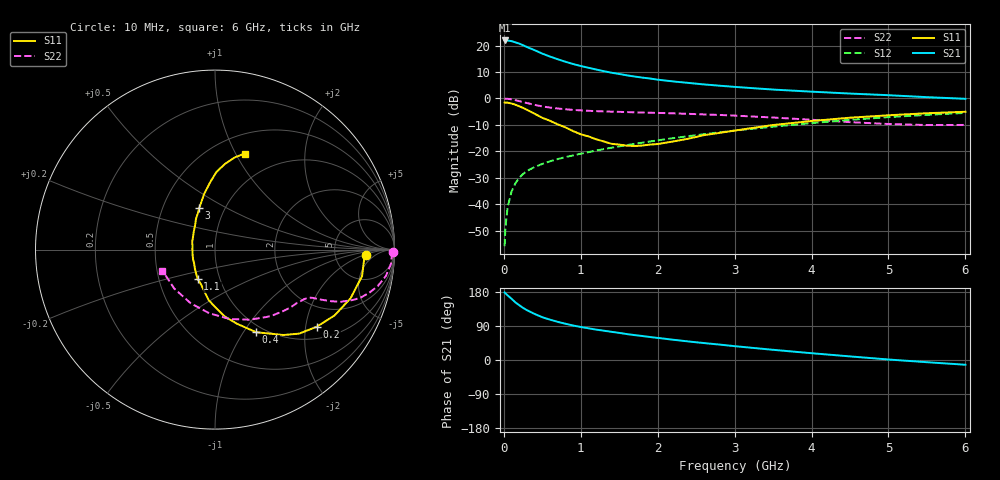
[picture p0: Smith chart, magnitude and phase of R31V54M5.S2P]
! SIEMENS Small Signal Semiconductors
! BFR181
! Si NPN RF Bipolar Junction Transistor in SOT23
! VCE = 1.5 V  IC = 4.5 mA
! Common Emitter S-Parameters:  May  1996
# GHz  S  MA  R  50
!  f  S11  S21  S12  S22
! GHz  MAG  ANG  MAG  ANG  MAG  ANG  MAG  ANG
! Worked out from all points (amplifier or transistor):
!   36 points, 10 MHz to 6 GHz, reference 50 ohm
!   highest |S21| = 22.0 dB at 10 MHz (marker M1)
!   |S21| within 3 dB of that: start of sweep to 343 MHz
!   unconditionally stable (mu >= 1): 1.082 GHz to 3.031 GHz
!   at 250 MHz: K = 0.40, MSG = 24.4 dB, |S12| = -28.6 dB
!   at 1.4 GHz: K = 1.06, MAG = 12.7 dB, |S12| = -18.7 dB
!   at 6 GHz: K = 0.87, MSG = 2.7 dB, |S12| = -5.5 dB
!   S11 on the Smith chart (normalised r, x): 10 MHz: 11, -2; 200 MHz: 1.33, -2.31; 400 MHz: 0.91, -1.14; 1.1 GHz: 0.78, -0.27; 3 GHz: 0.76, +0.37; 6 GHz: 0.70, +1.09
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0.01  0.8404 -2.1  12.53 178.2  0.0016 88.4  0.9909 -0.9
0.02  0.8323 -4.1  12.3 176.1  0.0036 85.0  0.9859 -1.8
0.05  0.8327 -10.2  12.49 170.5  0.0089 84.1  0.9839 -4.6
0.1  0.8024 -19.8  12.16 161.5  0.0173 80.1  0.9632 -8.8
0.15  0.7606 -28.8  11.52 152.1  0.0248 74.7  0.9298 -12.6
0.2  0.7118 -37.1  10.94 144.6  0.0314 71.7  0.8919 -15.7
0.25  0.663 -44.9  10.15 137.5  0.0372 68.1  0.8548 -18.2
0.3  0.6098 -51.3  9.415 131.5  0.0424 66.0  0.8198 -20.0
0.4  0.5137 -63.6  8.19 121.5  0.0504 63.1  0.7572 -22.6
0.5  0.4308 -73.5  7.057 112.8  0.0577 61.6  0.7067 -24.0
0.6  0.3781 -81.5  6.207 106.5  0.0647 61.3  0.6718 -24.8
0.7  0.3237 -89.2  5.526 100.7  0.0712 61.0  0.645 -25.5
0.9  0.2413 -104.1  4.486 91.0  0.0836 61.4  0.6072 -26.3
1.1  0.1915 -120.2  3.809 83.7  0.0963 62.3  0.5839 -27.5
1.3  0.1534 -137.0  3.278 77.3  0.11 62.5  0.5682 -29.0
1.6  0.1279 -167.9  2.737 68.4  0.131 62.6  0.5525 -31.9
2.2  0.1534 140.8  2.101 53.5  0.1772 61.5  0.5227 -39.2
3  0.2468 110.9  1.656 36.5  0.2458 57.0  0.4734 -52.4
3.5  0.314 101.3  1.473 26.9  0.2925 53.0  0.4357 -63.7
4.5  0.4322 89.0  1.238 9.5  0.393 42.6  0.3561 -95.1
5.5  0.5251 77.9  1.058 -5.8  0.4892 29.6  0.3141 -136.2
6  0.5597 72.9  0.985 -12.5  0.533 22.5  0.3153 -158.1
